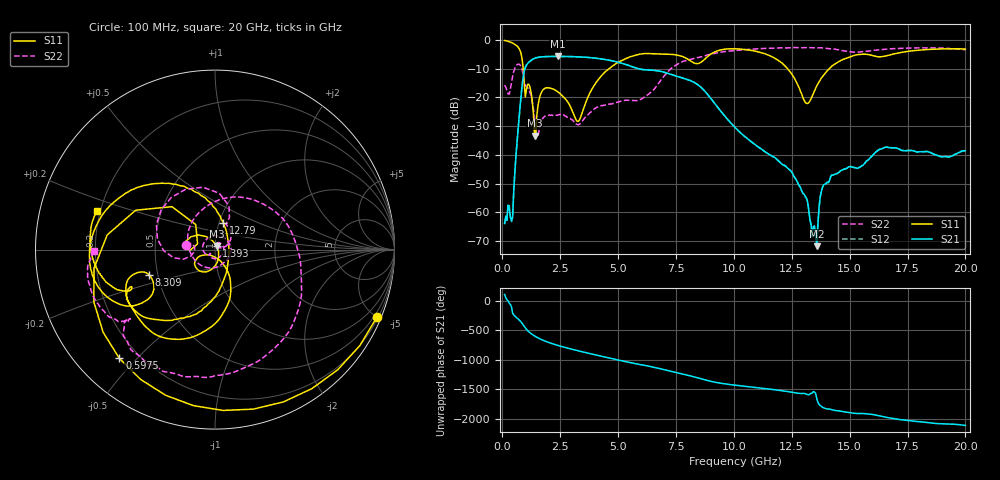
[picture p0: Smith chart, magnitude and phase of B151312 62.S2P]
!  2-Port S-parameters saved by WinCal
! VAR MeasName=S-Parameters (CALIBRATED_DATA) read from VNA (N5244A)
! VAR MeasDate=12/8/2015 5:48:38 PM
! VAR NAME=B151312 62
! VAR FILENAME=B151312 62.S2P
! VAR DATE=12/8/2015 5:48:38 PM
! VAR PHYS_PORTS=1,2
# Hz S DB R 50
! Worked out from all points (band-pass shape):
!   401 points, 100 MHz to 20 GHz, reference 50 ohm
!   highest |S21| = -5.75 dB at 2.389 GHz (marker M1); lowest = -71.7 dB at 13.58 GHz (marker M2)
!   |S21| within 3 dB of the highest: 1.044 GHz to 5.403 GHz (4.358 GHz wide, 135 % of centre)
!   lowest |S11| = -33.4 dB at 1.393 GHz (marker M3), VSWR 1.04, Z = 50.8 + j2 ohm
!   |S11| at or under -10 dB: 901.2 MHz to 4.61 GHz (3.709 GHz wide, 135 % of centre); 12.32 GHz to 14.12 GHz (1.799 GHz wide, 13.6 % of centre)
!   |S22| runs from -33.7 to -2.6 dB; largest |S21 - S12| = 0.0016
!   S11 on the Smith chart (normalised r, x): 100 MHz: 0.29, -4.99; 597.5 MHz: 0.13, -0.45; 1.393 GHz: 1.02, +0.04; 8.309 GHz: 0.45, -0.15; 12.79 GHz: 1.05, +0.32; 20 GHz: 0.19, +0.15
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1e8  -0.20 -22.6  -63.82 104.0  -64.03 107.4  -15.73 170.7
3.985e8  -0.94 -87.2  -62.93 -105.8  -63.20 -107.8  -14.77 -163.0
5.975e8  -1.86 -131.3  -39.54 78.8  -39.55 78.9  -9.00 156.9
9.4575e8  -15.09 127.6  -10.96 -76.4  -10.97 -76.5  -14.16 65.7
1.1945e9  -16.40 151.6  -7.43 176.3  -7.43 176.3  -18.22 42.6
1.3935e9  -33.35 65.9  -6.41 121.5  -6.41 121.5  -27.06 14.0
1.891e9  -16.67 -126.0  -5.81 27.7  -5.81 27.7  -26.40 37.5
2.3885e9  -17.99 -150.2  -5.75 -37.6  -5.74 -37.6  -26.22 -68.3
3.43325e9  -25.79 -75.6  -5.96 -145.0  -5.96 -145.0  -28.45 -139.2
4.72675e9  -9.28 -81.0  -7.26 97.7  -7.24 97.6  -22.26 90.4
5.62225e9  -5.62 -108.5  -9.36 21.7  -9.34 21.7  -21.06 -37.7
6.7665e9  -4.89 -140.4  -10.82 -69.4  -10.82 -69.5  -14.84 144.4
8.30875e9  -8.10 -159.3  -14.89 144.6  -14.86 144.4  -6.40 -7.4
1.005e10  -3.09 -177.2  -30.42 6.4  -30.39 5.8  -3.66 -64.9
1.1642e10  -5.85 134.2  -40.34 -64.4  -40.41 -64.5  -2.94 -97.1
1.278625e10  -16.13 72.4  -50.14 -130.5  -50.33 -130.3  -2.71 -115.1
1.338325e10  -19.56 -47.3  -68.42 -124.4  -68.39 -129.4  -2.74 -124.0
1.358225e10  -15.95 -69.5  -71.72 140.2  -69.56 135.2  -2.75 -127.5
1.3831e10  -12.78 -84.1  -51.26 -7.2  -50.97 -7.2  -2.80 -130.6
1.427875e10  -8.86 -104.7  -47.00 -54.4  -47.05 -54.2  -3.13 -137.3
1.67165e10  -5.31 -154.8  -37.48 171.8  -37.36 171.4  -3.12 -147.5
2e10  -3.19 162.0  -38.50 43.6  -38.68 43.2  -3.42 -179.5
